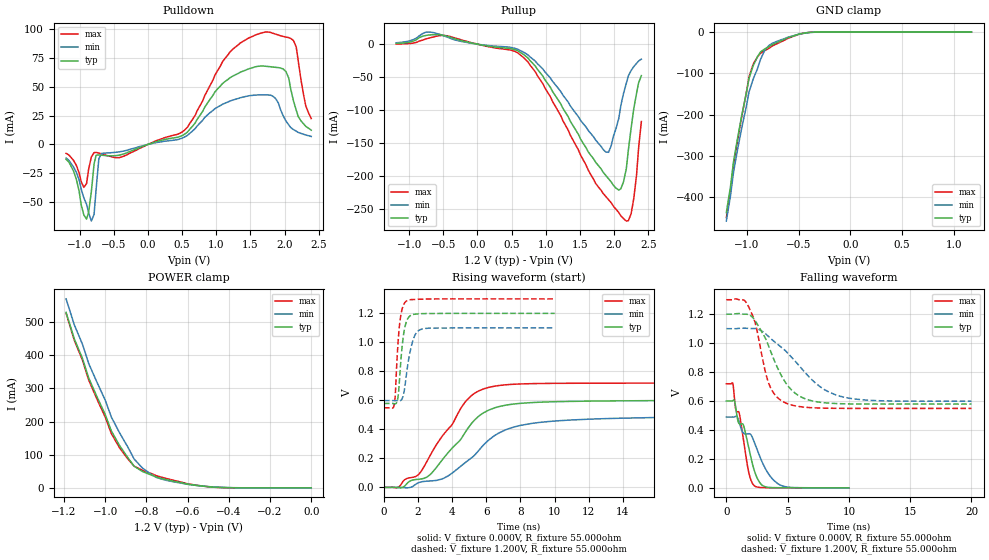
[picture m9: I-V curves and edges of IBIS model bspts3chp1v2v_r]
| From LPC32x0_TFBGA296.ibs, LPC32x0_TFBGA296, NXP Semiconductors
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| |   Rev 0.20 IBIS Model Design Automation Generation   |
| |   N O N - S I L I C O N   C O R R E L A T E D   |
| |   This IBIS [Model] is pre-Beta tactical support   |
| |  Note: this IBIS [Model] contains clamp curves generated   |
| |   through simulation which should not be relied upon   |
| bspts3chp1v2v
|   Bidirectional Pad 1v2
|   3state Output
|   Plain Input
|   3ns Slew Rate control
|   CMOS
|   Programmable between
|   - (p1=0, p2=1) plain input
|   - (p1=0, p2=0) with Pull Up
|   - (p1=1, p2=1) with Pull Down
|   - (p1=1, p2=0) with Repeater
|   Characterized at Core 1.2V and I/O 1.2V
| Repeater Mode (p1=1, p2=0)
[Model]   bspts3chp1v2v_r | of bspts3chp1v2v
Model_type   I/O
Polarity   Non-Inverting
Enable   Active-Low
|  Reciever Thresholds
Vinl   = 0.36V
Vinh   = 0.84V
| AC Test Load Conditions
Vref   = 0
Cref   = 1.2e-11
Rref   = 1000000000
Vmeas   = 0.6
| [Process Range]   typical   min   max
| C_comp edge width   400.000ps   400.000ps   400.000ps
| C_comp Tstrobe   40.000fs   40.000fs   40.000fs
C_comp   2.969pF   2.759pF   3.249pF
[Temperature Range]   25   105   -20
[Voltage Range]   1.20V   1.10V   1.30V
[GND Clamp Reference]   0.00V   0.00V   0.00V
[Pulldown Reference]   0.00V   0.00V   0.00V
[POWER Clamp Reference]   1.20V   1.10V   1.30V
[Pullup Reference]   1.20V   1.10V   1.30V
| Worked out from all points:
|   slope of the pulldown table from 0 to 0.18 V, typ, clamps not added: 55.1 ohm
|   slope of the pullup table from 0 to 0.18 V, typ, clamps not added: 53.4 ohm
|   GND clamp passes 1 mA (typ) near -0.40 V on its own axis
|   POWER clamp passes 1 mA (typ) near -0.43 V on its own axis
|   rising waveform, V_fixture 0.000V, R_fixture 55.000ohm: 20-80 % time 2.49ns typ, 3.01ns min, 2.32ns max; typ from 0 V to 0.599 V
|   falling waveform, V_fixture 0.000V, R_fixture 55.000ohm: 20-80 % time 1.38ns typ, 2.14ns min, 1.03ns max; typ from 0.6 V to 0 V
|   rising waveform, V_fixture 1.200V, R_fixture 55.000ohm: 20-80 % time 290ps typ, 433ps min, 251ps max; typ from 0.579 V to 1.2 V
|   falling waveform, V_fixture 1.200V, R_fixture 55.000ohm: 20-80 % time 2.13ns typ, 3.57ns min, 1.25ns max; typ from 1.2 V to 0.579 V
[GND Clamp]
| ref voltage   0.00V   0.00V   0.00V
|   Voltage   I(typ)   I(min)   I(max)
-1.2V     -437mA     -457.3mA   -448.8mA
-1.16V    -374mA     -396.6mA   -383.9mA
-1.13V    -313.1mA   -338.2mA   -320.9mA
-1.05V    -200.5mA   -230.7mA   -202.9mA
-980mV    -111.6mA   -144.4mA   -108mA
-940mV    -81.38mA   -113.4mA   -77.56mA
-870mV    -48.14mA   -66.68mA   -51.43mA
-830mV    -41.13mA   -44.64mA   -45.15mA
-790mV    -35.75mA   -33.05mA   -39.64mA
-570mV    -10.72mA   -10.13mA   -11.97mA
-390mV    -634.3uA   -1.09mA    -536.4uA
1.17V     -2.05uA    3.702uA    -9.85uA
[Power Clamp]   | Vtable = Vcc - Vpad
| ref voltage   1.20V   1.10V   1.30V
|   Voltage   I(typ)   I(min)   I(max)
-1.19V    529.3mA    570.1mA    526.5mA
-1.15V    449.5mA    491.7mA    445.3mA
-1.11V    389.5mA    432.5mA    384.2mA
-1.08V    331.1mA    374.7mA    324.8mA
-1V       221.2mA    264.5mA    213.3mA
-970mV    171.4mA    213.2mA    163.4mA
-890mV    91.03mA    122.9mA    86.98mA
-860mV    65.38mA    87.23mA    65.77mA
-820mV    49.53mA    60.17mA    53.08mA
-750mV    32.1mA     30.88mA    36.28mA
-560mV    7.554mA    7.588mA    8.109mA
0V        329.3nA    291.4nA    400.7nA
[Pulldown]
| ref voltage   0.00V   0.00V   0.00V
|   Voltage   I(typ)   I(min)   I(max)
-1.2V     -12.9mA    -11.81mA   -7.732mA
-900mV    -64.77mA   -51.94mA   -33.88mA
-830mV    -40.99mA   -66.41mA   -10.77mA
-760mV    -9.399mA   -38.71mA   -6.922mA
-720mV    -9.108mA   -12.33mA   -7.471mA
-680mV    -9.342mA   -7.831mA   -8.122mA
500mV     7.667mA    5.475mA    10.77mA
1.2V      57.8mA     37.61mA    80.16mA
1.72V     67.75mA    42.97mA    97.43mA
2.02V     63.13mA    20.22mA    93.1mA
2.13V     37.64mA    12.84mA    90mA
2.39V     12.34mA    6.89mA     22.38mA
[Pullup]   | Vtable = Vcc - Vpad
| ref voltage   1.20V   1.10V   1.30V
|   Voltage   I(typ)   I(min)   I(max)
-1.19V    982.9uA    2.112mA    262.9uA
-710mV    13.91mA    18.44mA    9.272mA
-450mV    12.25mA    11.02mA    12.78mA
590mV     -9.985mA   -7.698mA   -13.1mA
960mV     -48.84mA   -37.98mA   -60.41mA
1.88V     -199.3mA   -163.7mA   -231.3mA
1.96V     -209.3mA   -153.4mA   -241mA
2.07V     -221.5mA   -112.3mA   -255.7mA
2.18V     -188.8mA   -59.17mA   -268.4mA
2.25V     -127.4mA   -39.92mA   -257.5mA
2.33V     -74.27mA   -29.16mA   -198.1mA
2.4V      -47.76mA   -22.65mA   -117.4mA
[Ramp]
R_load   = 55.000ohm
|   dV/dt(typ)   dV/dt(min)   dV/dt(max)
dV/dt_r   337.978mV/2.450ns   259.332mV/2.715ns   412.738mV/2.315ns
dV/dt_f   356.319mV/2.195ns   272.300mV/3.335ns   433.855mV/1.325ns
[Rising Waveform]  | cubic spline decimation from 4001 points
V_fixture   = 0.000V
R_fixture   = 55.000ohm
|   Time   V(typ)   V(min)   V(max)
0s        162.8nV    2.485uV    161.4nV
755ps     -1.211mV   314.8uV    -2.713mV
1.945ns   55.04mV    27.45mV    80.76mV
2.63ns    80.36mV    43.51mV    203.3mV
3.51ns    203.6mV    63.23mV    367.7mV
4.735ns   374.7mV    168.1mV    584.4mV
5.85ns    515.1mV    294.2mV    679.5mV
7.16ns    567.3mV    398.4mV    707.6mV
9.11ns    587.2mV    447.8mV    716.2mV
20ns      599.4mV    486.2mV    719.2mV
[Falling Waveform]  | cubic spline decimation from 2001 points
V_fixture   = 0.000V
R_fixture   = 55.000ohm
|   Time   V(typ)   V(min)   V(max)
0s        600.3mV    489.5mV    719.4mV
520ps     601.5mV    489.6mV    723.2mV
755ps     562.7mV    494.4mV    549mV
1.055ns   442.8mV    451.9mV    516.2mV
1.4ns     432.2mV    377.6mV    331.5mV
1.815ns   282.8mV    373.9mV    112.8mV
2.29ns    117.5mV    313.4mV    13.8mV
2.96ns    15.79mV    170.8mV    1.945mV
4.385ns   881.1uV    19.75mV    309.4uV
10ns      7.647uV    93.44uV    1.443uV
[Rising Waveform]  | cubic spline decimation from 2001 points
V_fixture   = 1.200V
V_fixture_min = 1.100V
V_fixture_max = 1.300V
R_fixture   = 55.000ohm
|   Time   V(typ)   V(min)   V(max)
0s        578.8mV    598.5mV    549mV
600ps     577.2mV    598.5mV    567.7mV
670ps     576.5mV    598.5mV    651.5mV
800ps     607.5mV    597mV      950.3mV
925ps     765.2mV    596.4mV    1.134V
1.12ns    1.029V     628.5mV    1.251V
1.315ns   1.142V     775.9mV    1.285V
1.7ns     1.192V     1.014V     1.295V
2.16ns    1.198V     1.089V     1.298V
10ns      1.2V       1.1V       1.3V
[Falling Waveform]  | cubic spline decimation from 4001 points
V_fixture   = 1.200V
V_fixture_min = 1.100V
V_fixture_max = 1.300V
R_fixture   = 55.000ohm
|   Time   V(typ)   V(min)   V(max)
0s        1.2V       1.1V       1.3V
1.4ns     1.2V       1.103V     1.299V
1.77ns    1.199V     1.102V     1.26V
2.335ns   1.157V     1.101V     1.147V
3.47ns    975.6mV    1.044V     719.6mV
4.84ns    726.2mV    946.4mV    586.6mV
6.39ns    616.8mV    800.1mV    557.4mV
7.66ns    591.3mV    698.1mV    551.4mV
9.32ns    581.5mV    632.3mV    549.3mV
20ns      578.8mV    598.5mV    549mV
